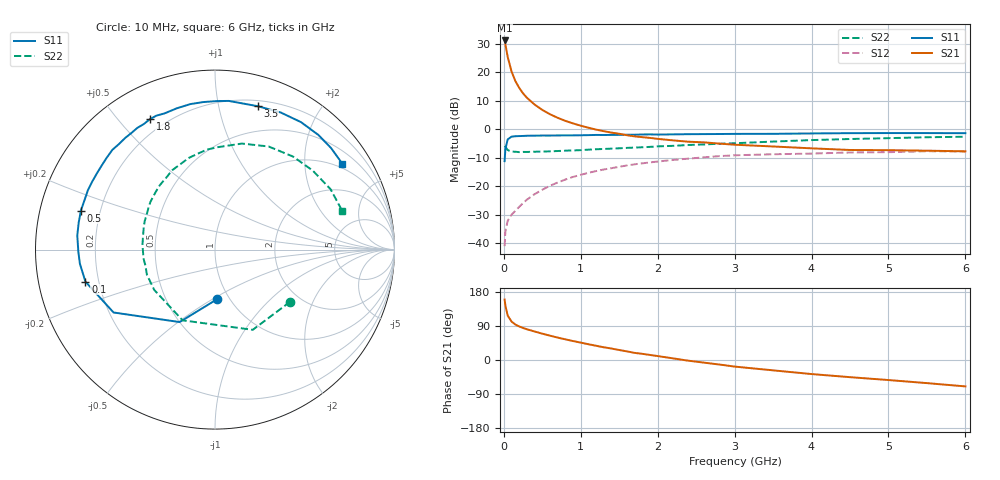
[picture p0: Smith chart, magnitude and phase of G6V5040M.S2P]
! SIEMENS Small Signal Semiconductors
! BFG193
! Si NPN RF Bipolar Junction Transistor in SOT223
! VCE = 0.5 V  IC = 40 mA
! Common Emitter S-Parameters:  August  1996
# GHz  S  MA  R  50
!  f  S11  S21  S12  S22
! GHz  MAG  ANG  MAG  ANG  MAG  ANG  MAG  ANG
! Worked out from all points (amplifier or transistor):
!   36 points, 10 MHz to 6 GHz, reference 50 ohm
!   highest |S21| = 31.2 dB at 10 MHz (marker M1)
!   |S21| within 3 dB of that: start of sweep to 31.42 MHz
!   unconditionally stable (mu >= 1): start of sweep to 11.43 MHz; 172.7 MHz to end of sweep
!   at 250 MHz: K = 1.12, MAG = 17.1 dB, |S12| = -25.9 dB
!   at 1.4 GHz: K = 1.23, MAG = 3.3 dB, |S12| = -13.6 dB
!   at 6 GHz: K = 1.07, MAG = -1.6 dB, |S12| = -7.8 dB
!   S11 on the Smith chart (normalised r, x): 10 MHz: 0.88, -0.52; 100 MHz: 0.15, -0.12; 500 MHz: 0.13, +0.14; 1.8 GHz: 0.14, +0.61; 3.5 GHz: 0.25, +1.31; 6 GHz: 0.85, +3.05
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0.01  0.2767 -87.6  36.29 159.6  0.0089 68.8  0.5095 -34.8
0.02  0.4492 -116.0  31.23 143.9  0.0161 58.6  0.494 -64.8
0.05  0.665 -148.2  18.7 117.2  0.0248 45.1  0.4334 -114.6
0.1  0.7435 -166.1  10.38 101.5  0.0317 44.4  0.4064 -146.5
0.15  0.7568 -174.0  7.022 93.5  0.0372 48.3  0.4043 -159.8
0.2  0.7612 -178.9  5.342 88.5  0.0437 52.4  0.3978 -167.2
0.25  0.7653 177.4  4.275 84.5  0.0509 54.0  0.4015 -173.2
0.3  0.7714 174.1  3.579 81.1  0.0583 56.0  0.401 -176.9
0.4  0.7742 168.8  2.72 75.2  0.0728 57.7  0.4049 176.2
0.5  0.7783 163.8  2.19 69.5  0.0872 57.3  0.4069 170.8
0.6  0.7774 159.3  1.84 64.2  0.1022 56.8  0.4107 166.5
0.7  0.7816 155.0  1.592 59.1  0.1167 55.2  0.4163 162.3
0.9  0.7834 146.9  1.27 50.0  0.1462 51.3  0.4262 154.0
1.1  0.7912 139.7  1.067 41.6  0.1723 47.0  0.4397 147.2
1.4  0.7983 128.9  0.875 30.2  0.2081 39.5  0.4586 136.8
1.8  0.8123 116.5  0.729 16.3  0.2532 29.5  0.4842 124.1
2.2  0.8155 105.1  0.64 4.3  0.2903 18.7  0.5131 112.2
3  0.8319 84.7  0.537 -17.4  0.3502 -1.4  0.5701 88.9
3.5  0.8337 73.4  0.5 -27.3  0.3651 -14.6  0.6097 75.7
4.5  0.8567 56.0  0.434 -45.3  0.3923 -33.2  0.6766 50.0
5.5  0.8593 41.2  0.422 -61.0  0.4127 -54.3  0.7265 27.6
6  0.8558 34.0  0.411 -69.7  0.4073 -66.3  0.7408 17.0
